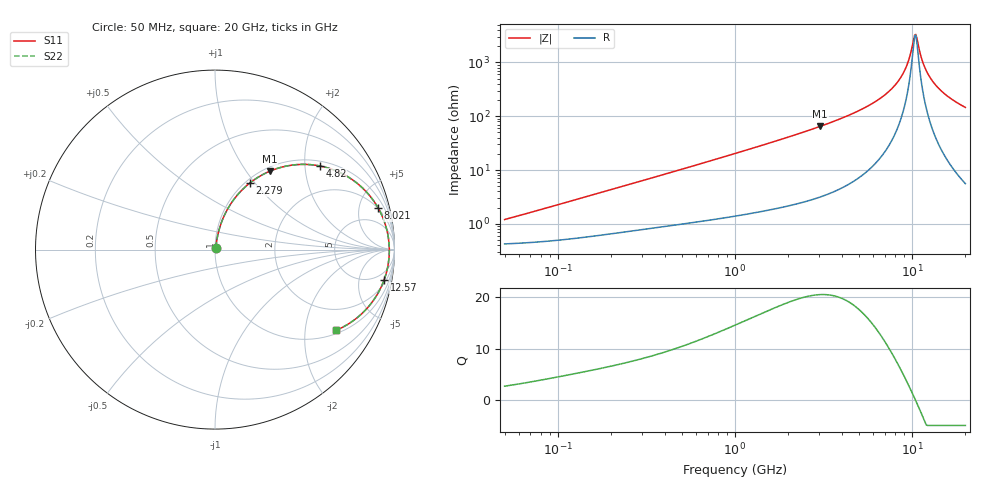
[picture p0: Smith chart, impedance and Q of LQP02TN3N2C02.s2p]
!Murata Part Number: LQP02TN3N2C02
!These Parameters are Measured in Series Mode Connection
!  o--[Z]--o
!Port1  Port2
!  o-------o
!Freq. Start=50[MHz] Stop=20[GHz], 401[Steps]
# Hz S RI R 50
!Freq.(Hz) S11(Real) S11(Imag) S21(Real) S21(Imag) S12(Real) S12(Imag) S22(Real) S22(Imag)
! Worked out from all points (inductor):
!   401 points, 50 MHz to 20 GHz, reference 50 ohm
!   read as one part in series: L = 3.56 nH near 58.08 MHz
!   highest Q = 20.5 at 3.03 GHz (marker M1), where L = 3.41 nH
!   self-resonance near 10.35 GHz
!   S11 on the Smith chart (normalised r, x): 50 MHz: 1.01, +0.02; 2.279 GHz: 1.05, +0.94; 4.82 GHz: 1.13, +2.39; 8.021 GHz: 1.95, +7.53; 12.57 GHz: 3, -11; 20 GHz: 1.11, -2.91
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5e7  0.00435 0.0112  0.9956 -0.0112  0.9956 -0.0112  0.00435 0.0112
1.364002e8  0.00641 0.0295  0.9936 -0.0295  0.9936 -0.0295  0.00641 0.0295
3.721004e8  0.0144 0.0757  0.9856 -0.0757  0.9856 -0.0757  0.0144 0.0757
1e9  0.0515 0.1893  0.9485 -0.1893  0.9485 -0.1893  0.0515 0.1893
2.279204e9  0.1939 0.3708  0.8061 -0.3708  0.8061 -0.3708  0.1939 0.3708
2.728004e9  0.2589 0.4141  0.7411 -0.4141  0.7411 -0.4141  0.2589 0.4141
3.029571e9  0.305 0.4367  0.695 -0.4367  0.695 -0.4367  0.305 0.4367
4.81993e9  0.5841 0.466  0.4159 -0.466  0.4159 -0.466  0.5841 0.466
6.125241e9  0.7533 0.3976  0.2467 -0.3976  0.2467 -0.3976  0.7533 0.3976
7.442007e9  0.8735 0.2858  0.1265 -0.2858  0.1265 -0.2858  0.8735 0.2858
8.020766e9  0.9098 0.2304  0.0902 -0.2304  0.0902 -0.2304  0.9098 0.2304
8.644534e9  0.9387 0.1693  0.0613 -0.1693  0.0613 -0.1693  0.9387 0.1693
9.178299e9  0.9555 0.1172  0.0445 -0.1172  0.0445 -0.1172  0.9555 0.1172
9.600142e9  0.9643 0.0768  0.0357 -0.0768  0.0357 -0.0768  0.9643 0.0768
1.019291e10  0.9705 0.0218  0.0295 -0.0218  0.0295 -0.0218  0.9705 0.0218
1.034674e10  0.971 0.00795  0.029 -0.00795  0.029 -0.00795  0.971 0.00795
1.066139e10  0.971 -0.0198  0.029 0.0198  0.029 0.0198  0.971 -0.0198
1.149051e10  0.9638 -0.0888  0.0362 0.0888  0.0362 0.0888  0.9638 -0.0888
1.257102e10  0.9424 -0.1687  0.0576 0.1687  0.0576 0.1687  0.9424 -0.1687
1.375312e10  0.9081 -0.2428  0.0919 0.2428  0.0919 0.2428  0.9081 -0.2428
1.527346e10  0.8544 -0.3191  0.1456 0.3191  0.1456 0.3191  0.8544 -0.3191
2e10  0.6736 -0.4501  0.3264 0.4501  0.3264 0.4501  0.6736 -0.4501
